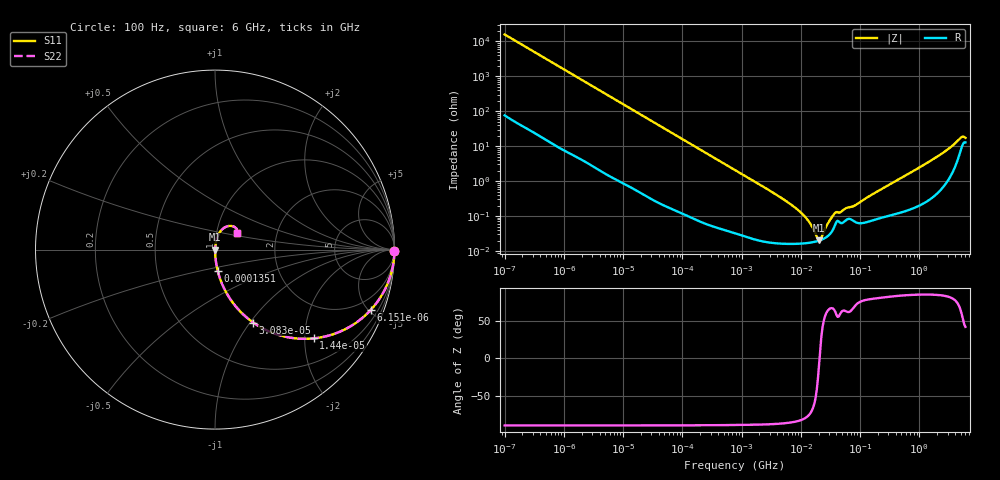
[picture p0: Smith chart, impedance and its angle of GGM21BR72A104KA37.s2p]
!Murata Part Number: GGM21BR72A104KA37
!These Parameters are Measured in Series Mode Connection
!Data Generated on Jun 19, 2026
!  o--ll--o
!Port1  Port2
!  o------o
!Operation Temp=25[degC], DC Bias Voltage=0[V]
!Freq. Start=100[Hz] Stop=6[GHz] 401[Steps]
# Hz S RI R 50
!Freq.(Hz) S11(Real) S11(Imag) S21(Real) S21(Imag) S12(Real) S12(Imag) S22(Real) S22(Imag)
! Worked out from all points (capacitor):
!   401 points, 100 Hz to 6 GHz, reference 50 ohm
!   read as one part in series: C = 101 nF near 109 Hz
!   lowest |Z| = 20.1 mohm at 20.35 MHz (marker M1)
!   series resonance near 20.68 MHz, so ESL is about 590 pH
!   S11 on the Smith chart (normalised r, x): 100 Hz: open; 6.151 kHz: 1.03, -5.17; 14.4 kHz: 1.01, -2.21; 30.83 kHz: 1.01, -1.04; 135.1 kHz: 1.00, -0.24; 6 GHz: 1.26, +0.23
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100  0.9999 -0.00637  7.15e-05 0.00637  7.15e-05 0.00637  0.9999 -0.00637
627  0.9982 -0.0396  0.00176 0.0396  0.00176 0.0396  0.9982 -0.0396
2008  0.9836 -0.1246  0.0164 0.1246  0.0164 0.1246  0.9836 -0.1246
6151  0.8685 -0.3354  0.1315 0.3354  0.1315 0.3354  0.8685 -0.3354
14402  0.5503 -0.4947  0.4497 0.4947  0.4497 0.4947  0.5503 -0.4947
30832  0.2132 -0.4067  0.7868 0.4067  0.7868 0.4067  0.2132 -0.4067
40335  0.1374 -0.3413  0.8626 0.3413  0.8626 0.3413  0.1374 -0.3413
135116  0.0148 -0.1171  0.9852 0.1171  0.9852 0.1171  0.0148 -0.1171
774597  0.000759 -0.0209  0.9992 0.0209  0.9992 0.0209  0.000759 -0.0209
6948629  0.000164 -0.00209  0.9998 0.00209  0.9998 0.00209  0.000164 -0.00209
1.137099e7  0.000167 -0.00101  0.9998 0.00101  0.9998 0.00101  0.000167 -0.00101
1.555665e7  0.000178 -0.000461  0.9998 0.000461  0.9998 0.000461  0.000178 -0.000461
1.86079e7  0.00019 -0.00017  0.9998 0.00017  0.9998 0.00017  0.00019 -0.00017
2.035112e7  0.000199 -2.55e-05  0.9998 2.55e-05  0.9998 2.55e-05  0.000199 -2.55e-05
2.225763e7  0.00021 0.00012  0.9998 -0.00012  0.9998 -0.00012  0.00021 0.00012
2.911731e7  0.000275 0.000586  0.9997 -0.000586  0.9997 -0.000586  0.000275 0.000586
3.80911e7  0.000573 0.0011  0.9994 -0.0011  0.9994 -0.0011  0.000573 0.0011
8.154455e7  0.00069 0.00189  0.9993 -0.00189  0.9993 -0.00189  0.00069 0.00189
3.124326e8  0.00109 0.00779  0.9989 -0.00779  0.9989 -0.00779  0.00109 0.00779
1.95892e9  0.0066 0.0483  0.9934 -0.0483  0.9934 -0.0483  0.0066 0.0483
5.016141e9  0.0908 0.1322  0.9092 -0.1322  0.9092 -0.1322  0.0908 0.1322
6e9  0.1229 0.0904  0.8771 -0.0904  0.8771 -0.0904  0.1229 0.0904
